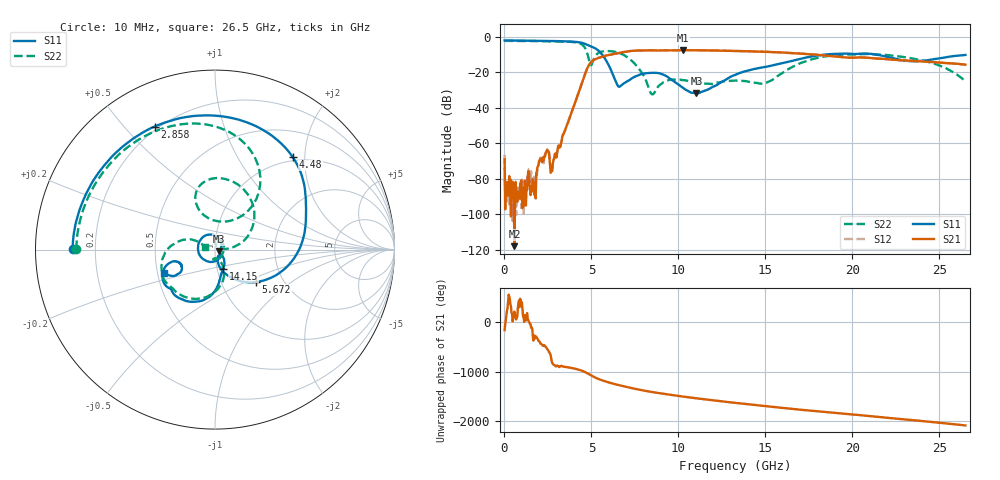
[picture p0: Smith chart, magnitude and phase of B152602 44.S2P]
!  2-Port S-parameters saved by WinCal
! VAR MeasName=S-Parameters (CALIBRATED_DATA) read from VNA (N5242A)
! VAR MeasDate=2016-1-5 16:32:28
! VAR NAME=B152602 44
! VAR FILENAME=B152602 44.S2P
! VAR DATE=2016-1-5 16:32:28
! VAR PHYS_PORTS=1,2
# Hz S DB R 50
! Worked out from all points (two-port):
!   801 points, 10 MHz to 26.5 GHz, reference 50 ohm
!   highest |S21| = -7.48 dB at 10.27 GHz (marker M1); lowest = -118.0 dB at 572.9 MHz (marker M2)
!   |S21| within 3 dB of the highest: 5.867 GHz to 18.41 GHz (12.54 GHz wide, 103 % of centre)
!   lowest |S11| = -31.8 dB at 11.04 GHz (marker M3), VSWR 1.05, Z = 52.4 - j1.1 ohm
!   |S11| at or under -10 dB: 5.618 GHz to 18.42 GHz (12.8 GHz wide, 107 % of centre); 21.39 GHz to end of sweep
!   |S22| runs from -32.4 to -2.2 dB; largest |S21 - S12| = 0.0032
!   S11 on the Smith chart (normalised r, x): 10 MHz: 0.12, +0.00; 2.858 GHz: 0.18, +0.61; 4.48 GHz: 0.93, +1.76; 5.672 GHz: 1.46, -0.58; 14.15 GHz: 1.07, -0.23; 26.5 GHz: 0.54, -0.16
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1e7  -2.01 179.7  -69.05 -160.2  -66.53 -22.7  -2.24 179.8
1.755625e8  -2.02 176.3  -81.83 -79.3  -94.18 120.5  -2.25 177.3
5.729125e8  -2.06 168.2  -117.95 -145.7  -94.97 -173.4  -2.27 171.1
1.73185e9  -2.21 143.9  -89.11 91.2  -84.67 92.5  -2.36 152.8
2.427212e9  -2.29 127.6  -64.36 -164.3  -64.53 -160.5  -2.44 140.5
2.725225e9  -2.32 119.8  -75.59 -84.3  -75.21 -89.0  -2.46 134.7
2.857675e9  -2.34 116.1  -68.69 -147.4  -68.99 -152.6  -2.49 131.9
4.447075e9  -3.36 51.9  -26.14 100.3  -26.14 100.6  -4.25 74.2
4.480188e9  -3.44 49.9  -25.17 96.1  -25.18 96.2  -4.49 71.6
4.976875e9  -5.37 19.9  -14.32 3.7  -14.32 3.8  -16.00 83.5
5.672238e9  -10.71 -38.2  -11.00 -102.1  -10.99 -102.0  -8.15 95.2
6.599388e9  -28.14 -58.1  -8.99 165.6  -8.99 165.7  -9.07 57.4
7.493425e9  -22.47 -116.0  -7.76 93.7  -7.75 93.8  -15.15 18.1
8.453688e9  -20.22 156.5  -7.60 30.3  -7.60 30.3  -32.12 40.2
8.851038e9  -20.39 126.1  -7.65 7.8  -7.65 7.7  -27.82 90.8
1.027488e10  -28.79 17.9  -7.48 -64.5  -7.49 -64.5  -24.39 59.0
1.103646e10  -31.82 -24.1  -7.56 -99.6  -7.56 -99.5  -25.35 24.4
1.3255e10  -21.43 -52.4  -7.94 169.1  -7.93 169.1  -24.61 -87.2
1.414904e10  -18.64 -67.0  -8.16 134.7  -8.12 134.8  -25.53 -100.1
1.769208e10  -10.96 -101.3  -9.86 6.2  -9.82 6.3  -12.58 -90.1
2.209604e10  -11.42 -163.3  -12.67 -136.7  -12.64 -137.1  -10.34 -166.9
2.65e10  -10.17 -155.2  -15.66 71.4  -15.67 71.2  -24.91 166.1
